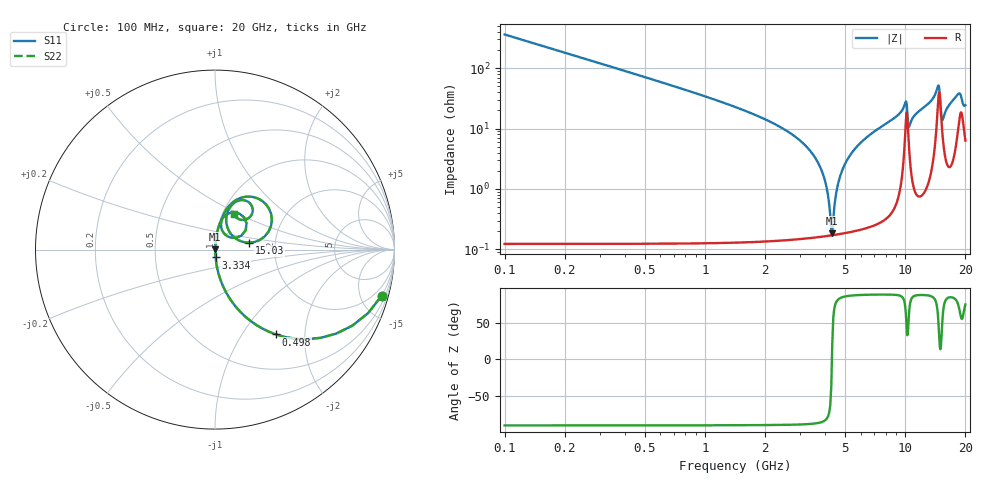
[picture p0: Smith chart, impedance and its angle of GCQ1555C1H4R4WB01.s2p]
!Murata Part Number: GCQ1555C1H4R4WB01
!These Parameters are Measured in Series Mode Connection
!Data Generated on Jan 08, 2026
!  o--ll--o
!Port1  Port2
!  o------o
!Operation Temp=25[degC], DC Bias Voltage=0[V]
!Freq. Start=100[MHz] Stop=20[GHz] 401[Steps]
# Hz S RI R 50
!Freq.(Hz) S11(Real) S11(Imag) S21(Real) S21(Imag) S12(Real) S12(Imag) S22(Real) S22(Imag)
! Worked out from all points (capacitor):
!   401 points, 100 MHz to 20 GHz, reference 50 ohm
!   read as one part in series: C = 4.4 pF near 199.5 MHz
!   lowest |Z| = 185 mohm at 4.329 GHz (marker M1)
!   series resonance near 4.311 GHz, so ESL is about 310 pH
!   S11 on the Smith chart (normalised r, x): 100 MHz: 1.00, -7.23; 498 MHz: 1.00, -1.43; 3.334 GHz: 1.00, -0.09; 15.03 GHz: 1.47, +0.12; 20 GHz: 1.13, +0.47
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1e8  0.9289 -0.2569  0.0711 0.2569  0.0711 0.2569  0.9289 -0.2569
4.98e8  0.3396 -0.4727  0.6604 0.4727  0.6604 0.4727  0.3396 -0.4727
1.24425e9  0.0675 -0.2484  0.9325 0.2484  0.9325 0.2484  0.0675 -0.2484
3.33375e9  0.00345 -0.0437  0.9966 0.0437  0.9966 0.0437  0.00345 -0.0437
3.43325e9  0.00305 -0.0387  0.997 0.0387  0.997 0.0387  0.00305 -0.0387
3.93075e9  0.00188 -0.0156  0.9981 0.0156  0.9981 0.0156  0.00188 -0.0156
4.08e9  0.00175 -0.00932  0.9983 0.00932  0.9983 0.00932  0.00175 -0.00932
4.22925e9  0.0017 -0.00323  0.9983 0.00323  0.9983 0.00323  0.0017 -0.00323
4.32875e9  0.00171 0.000707  0.9983 -0.000707  0.9983 -0.000707  0.00171 0.000707
4.62725e9  0.00192 0.0121  0.9981 -0.0121  0.9981 -0.0121  0.00192 0.0121
5.02525e9  0.00255 0.0262  0.9975 -0.0262  0.9975 -0.0262  0.00255 0.0262
6.7665e9  0.00898 0.0809  0.991 -0.0809  0.991 -0.0809  0.00898 0.0809
1.005e10  0.1398 0.1983  0.8602 -0.1983  0.8602 -0.1983  0.1398 0.1983
1.0448e10  0.0569 0.0835  0.9431 -0.0835  0.9431 -0.0835  0.0569 0.0835
1.1244e10  0.0361 0.1625  0.9639 -0.1625  0.9639 -0.1625  0.0361 0.1625
1.338325e10  0.0857 0.2513  0.9143 -0.2513  0.9143 -0.2513  0.0857 0.2513
1.4627e10  0.2998 0.2301  0.7002 -0.2301  0.7002 -0.2301  0.2998 0.2301
1.5025e10  0.1911 0.0384  0.8089 -0.0384  0.8089 -0.0384  0.1911 0.0384
1.53235e10  0.0898 0.0863  0.9102 -0.0863  0.9102 -0.0863  0.0898 0.0863
1.67165e10  0.0789 0.2279  0.9211 -0.2279  0.9211 -0.2279  0.0789 0.2279
1.85075e10  0.1883 0.2636  0.8117 -0.2636  0.8117 -0.2636  0.1883 0.2636
2e10  0.1034 0.1987  0.8966 -0.1987  0.8966 -0.1987  0.1034 0.1987
